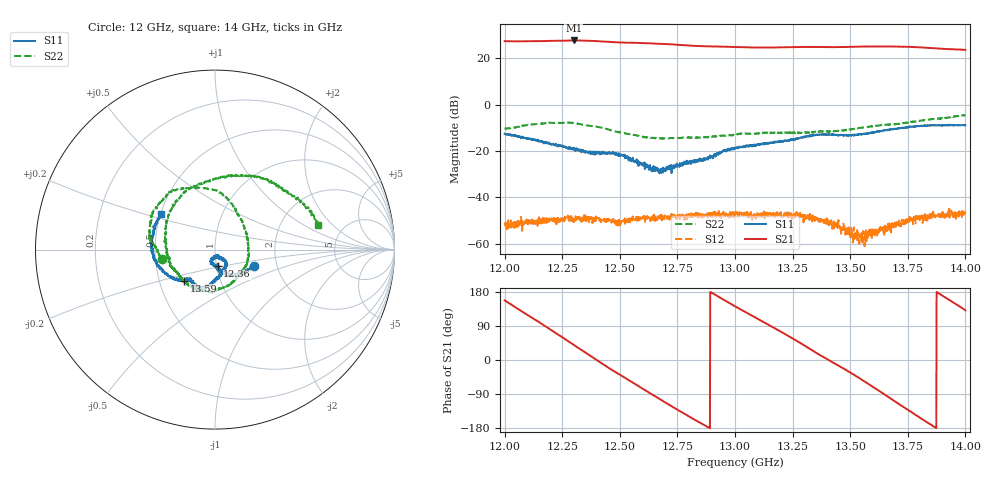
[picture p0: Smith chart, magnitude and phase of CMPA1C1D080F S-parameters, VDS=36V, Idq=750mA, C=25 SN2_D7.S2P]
!Keysight Technologies,E5071C,MY46632380,B.14.03
!Date: Thu Nov 05 05:03:59 2020
!Data & Calibration Information:
!Freq	S11:SOLT2(ON)	S21:SOLT2(ON)	S12:SOLT2(ON)	S22:SOLT2(ON)
!PortZ  Port1:50+j0  Port2:50+j0
!Above PortZ is port z conversion or system Z0 setting when saving the data.
!When reading, reference impedance value at option line is always used.
# Hz S dB R 50
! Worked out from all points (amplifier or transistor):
!   1601 points, 12 GHz to 14 GHz, reference 50 ohm
!   highest |S21| = 27.6 dB at 12.3 GHz (marker M1)
!   |S21| within 3 dB of that: start of sweep to 13.07 GHz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
!   unconditionally stable (mu >= 1): start of sweep to end of sweep
!   at 12.33 GHz: K = 5.43, MAG = 28.2 dB, |S12| = -49.5 dB
!   at 13 GHz: K = 6.39, MAG = 25.1 dB, |S12| = -47.4 dB
!   at 14 GHz: K = 4.51, MAG = 26.0 dB, |S12| = -47.5 dB
!   S11 on the Smith chart (normalised r, x): 12 GHz: 1.52, -0.29; 12.36 GHz: 1.01, -0.19; 13.59 GHz: 0.67, -0.25; 14 GHz: 0.50, +0.23
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1.2e10  -12.63 -22.3  27.30 157.4  -52.12 -131.6  -10.43 -169.8
1.208875e10  -14.54 -45.6  27.25 123.0  -50.24 -131.0  -8.93 173.7
1.216e10  -15.69 -60.5  27.31 95.6  -51.24 -139.3  -8.18 157.8
1.22275e10  -17.81 -71.8  27.47 69.0  -49.10 -141.1  -7.89 140.7
1.23e10  -19.45 -85.9  27.60 40.0  -50.71 -143.2  -8.05 123.1
1.233375e10  -20.62 -87.3  27.56 26.5  -50.58 -146.3  -8.67 113.1
1.236e10  -20.62 -80.8  27.49 15.8  -48.51 -163.2  -9.00 104.2
1.243625e10  -20.62 -87.7  27.10 -14.8  -49.47 -178.1  -10.48 79.9
1.253125e10  -22.28 -108.1  26.63 -50.2  -49.37 -179.6  -12.64 57.3
1.259875e10  -25.87 -104.4  26.51 -75.5  -48.72 175.1  -13.88 33.7
1.26675e10  -27.89 -85.8  26.18 -100.9  -48.67 169.3  -14.48 11.6
1.283125e10  -24.52 -53.0  25.26 -159.8  -47.34 142.4  -14.34 -36.7
1.292125e10  -21.59 -49.3  25.01 169.8  -47.60 129.0  -13.69 -61.9
1.3e10  -18.81 -61.4  24.77 141.7  -47.44 109.4  -12.95 -86.8
1.317375e10  -16.28 -81.1  24.58 83.3  -48.47 82.8  -12.30 -122.3
1.333375e10  -13.24 -104.4  24.80 25.9  -49.06 42.6  -11.80 -154.9
1.346e10  -12.92 -126.8  24.75 -18.8  -55.66 1.8  -11.14 175.9
1.3585e10  -12.15 -134.8  24.98 -65.7  -55.25 21.0  -9.49 136.8
1.36675e10  -10.96 -147.0  25.00 -98.4  -52.86 42.5  -8.62 109.7
1.38275e10  -9.06 -178.5  24.45 -161.9  -47.61 7.9  -6.65 61.7
1.3905e10  -8.98 163.5  23.96 167.9  -47.30 -33.6  -5.99 41.2
1.4e10  -8.89 146.5  23.54 130.9  -47.50 -60.2  -4.59 13.5
